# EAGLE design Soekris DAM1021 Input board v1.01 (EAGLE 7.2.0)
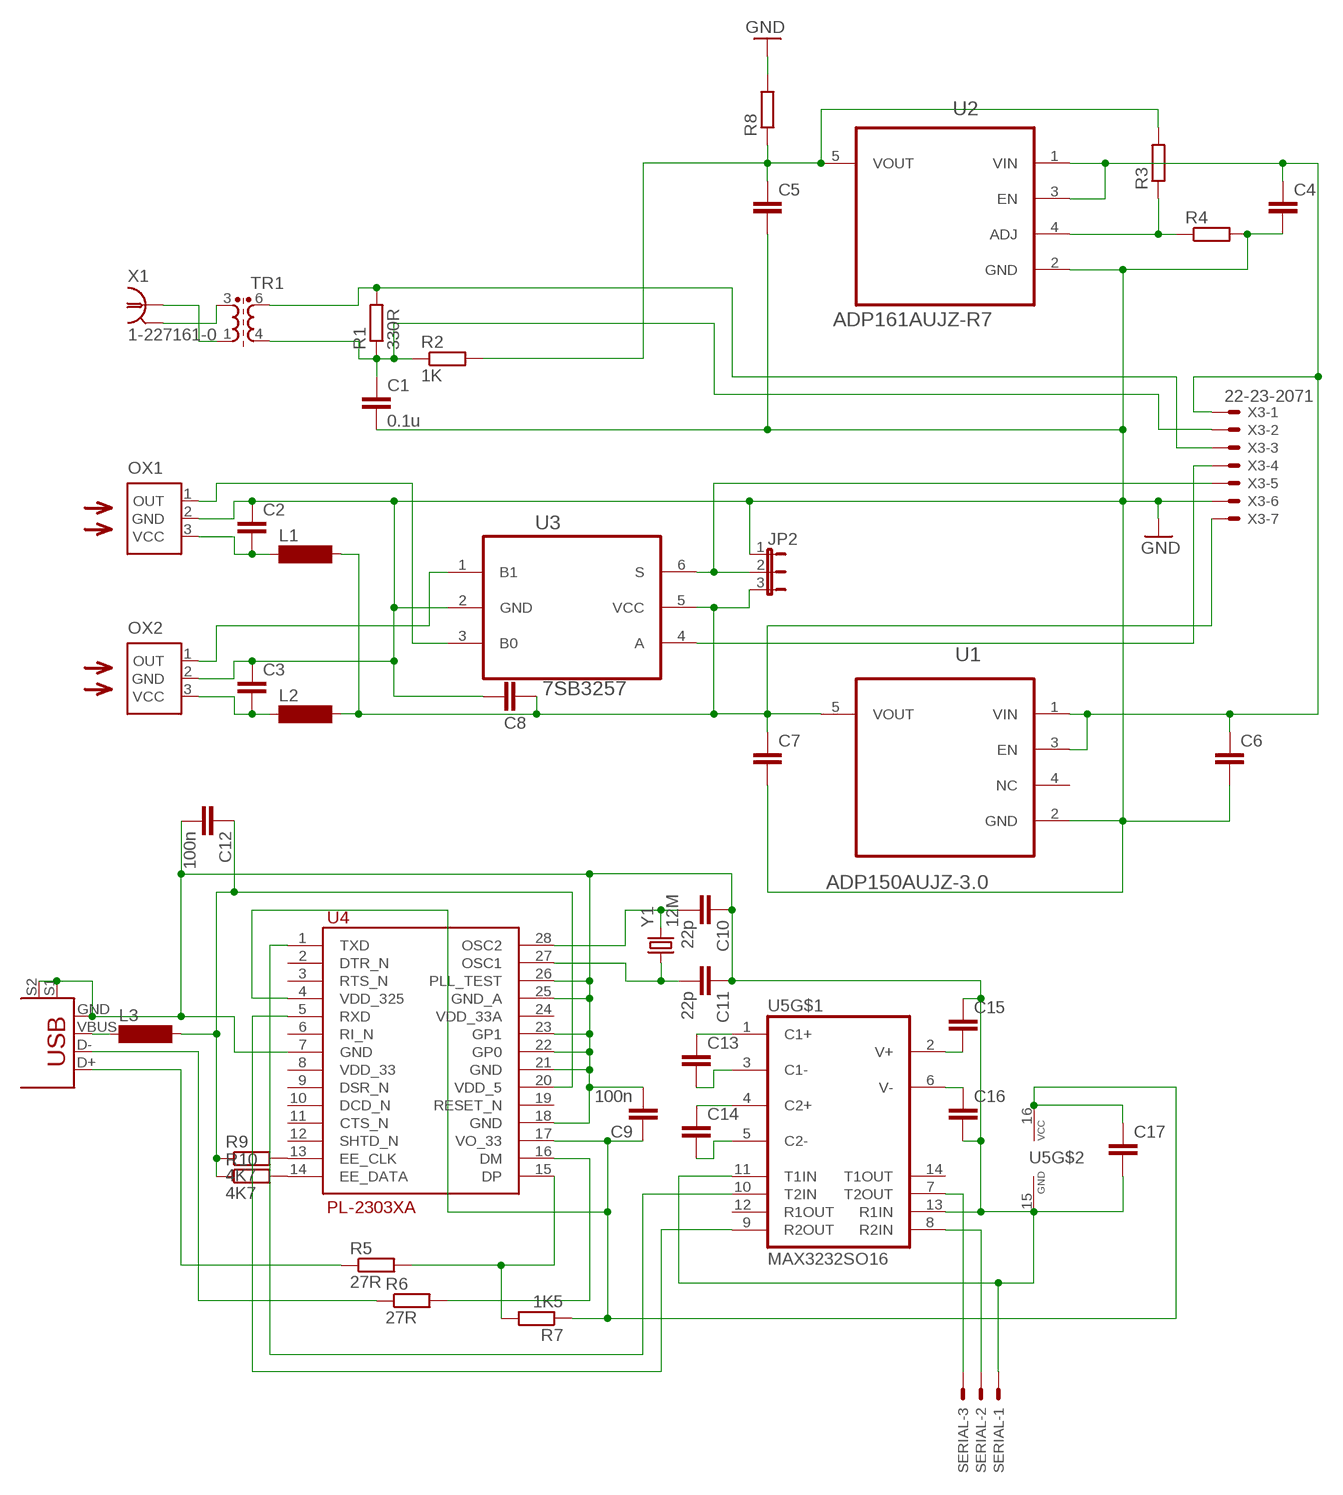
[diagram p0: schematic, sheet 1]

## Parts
C1  0.1u  C-EUC0805  [C0805]
C2  C-EUC0805  [C0805]
C3  C-EUC0805  [C0805]
C4  C-EUC1206  [C1206]
C5  C-EUC1206  [C1206]
C6  C-EUC1206  [C1206]
C7  C-EUC1206  [C1206]
C8  C-EUC1206  [C1206]
C9  100n  C-EUC1206  [C1206]
C10  22p  C-EUC1206  [C1206]
C11  22p  C-EUC1206  [C1206]
C12  100n  C-EUC1206  [C1206]
C13  C-EUC1206  [C1206]
C14  C-EUC1206  [C1206]
C15  C-EUC1206  [C1206]
C16  C-EUC1206  [C1206]
C17  C-EUC1206  [C1206]
JP2  JP2E  [JP2]
L1  SM-1206  [SM-1206]
L2  SM-1206  [SM-1206]
L3  SM-1206  [SM-1206]
OX1  TORX177(F,T)  [TORX]
OX2  TORX177(F,T)  [TORX]
R1  330R  R-EU_R0805  [R0805]
R2  1K  R-EU_R1206  [R1206]
R3  R-EU_R1206  [R1206]
R4  R-EU_R1206  [R1206]
R5  27R  R-EU_M1206  [M1206]
R6  27R  R-EU_M1206  [M1206]
R7  1K5  R-EU_M0805  [M0805]
R8  R-EU_R0805  [R0805]
R9  4K7  R-EU_M0805  [M0805]
R10  4K7  R-EU_M0805  [M0805]
SERIAL  22-23-2031  [22-23-2031]
TR1  DA101C  [DA101C]
U1  ADP150AUJZ-3.0  [SOT95P280X100-5N]
U2  ADP161AUJZ-R7  [SOT95P280X100-5N]
U3  7SB3257  [TSOP-6]
U4  PL-2303XA  [SSOP28]
U5  MAX3232SO16  [SO16]
USB  USB+SHIELD  [USB-B-PTH]
X1  1-227161-0  [AMP_227161]
X3  22-23-2071  [22-23-2071]
Y1  12M  CRYSTALHC49US  [HC49US]

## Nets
GND: C1.2 C2.1 C3.1 C4.2 C5.2 C6.2 C7.2 C8.1 JP2.1 OX1.2(GND) OX2.2(GND) R4.2 R8.2 U1.2(GND) U2.2(GND) U3.2(GND) X3.6
N$1: C4.1 C6.1 U1.1(VIN) U1.3(EN) U2.1(VIN) U2.3(EN) X3.1
N$2: C2.2 L1.1 OX1.3(VCC)
N$3: R3.1 R4.1 U2.4(ADJ)
N$4: C3.2 L2.1 OX2.3(VCC)
N$5: TR1.1 X1.1
N$6: TR1.3 X1.2
N$7: R1.2 TR1.6 X3.3
N$8: C1.1 R1.1 R2.1 TR1.4 X3.2
N$9: C9.1 C17.1 R7.1 U4.4(VDD_325) U4.17(VO_33) U5.16(VCC)
N$10: OX2.1(OUT) U3.1(B1)
N$11: OX1.1(OUT) U3.3(B0)
N$12: C7.1 C8.2 JP2.3 L1.2 L2.2 U1.5(VOUT) U3.5(VCC) X3.7
N$13: JP2.2 U3.6(S) X3.5
N$14: C5.1 R2.2 R3.2 R8.1 U2.5(VOUT)
N$15: R9.2 U4.13(EE_CLK)
N$16: L3.1 USB.VBUS
N$17: U3.4(A) X3.4
N$18: R5.2 R7.2 U4.15(DP)
N$19: R6.2 U4.16(DM)
N$20: R6.1 USB.D-
N$21: R5.1 USB.D+
N$22: C10.2 U4.28(OSC2) Y1.2
N$23: C11.2 U4.27(OSC1) Y1.1
N$24: R10.2 U4.14(EE_DATA)
N$25: C12.1 L3.2 R9.1 R10.1 U4.20(VDD_5)
N$27: SERIAL.2 U5.8(R2IN)
N$28: C13.1 U5.1(C1+)
N$29: C13.2 U5.3(C1-)
N$30: C14.1 U5.4(C2+)
N$31: C14.2 U5.5(C2-)
N$32: C15.2 U5.2(V+)
N$33: C16.1 U5.6(V-)
N$34: C9.2 C10.1 C11.1 C12.2 C15.1 C16.2 C17.2 SERIAL.1 U4.7(GND) U4.18(GND) U4.21(GND) U4.22(GP0) U4.23(GP1) U4.25(GND_A) U4.26(PLL_TEST) U5.11(T1IN) U5.13(R1IN) U5.15(GND2) USB.GND USB.S1 USB.S2
N$37: U4.1(TXD) U5.10(T2IN)
N$38: SERIAL.3 U5.7(T2OUT)
N$40: U4.5(RXD) U5.9(R2OUT)
Unconnected: U1.4(NC) U4.2(DTR_N) U4.3(RTS_N) U4.6(RI_N) U4.8(VDD_33) U4.9(DSR_N) U4.10(DCD_N) U4.11(CTS_N) U4.12(SHTD_N) U4.19(RESET_N) U4.24(VDD_33A) U5.12(R1OUT) U5.14(T1OUT)

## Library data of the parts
C1-C17 = rcl:C-EU: CAPACITOR, European symbol
JP2 = jumper:JP2E: JUMPER
L1-L3 = inductor-neosid:SM-1206: INDUCTOR; OC_FARNELL: unknown; OC_NEWARK: unknown
OX1 OX2 = dir9001_spdif12:TORX177(F,T): FIBER OPTIC RECEIVING MODULE
R1-R10 = rcl:R-EU_: RESISTOR, European symbol
SERIAL = con-molex:22-23-2031: .100" (2.54mm) Center Header - 3 Pin; MF: MOLEX; MPN: 22-23-2031; OC_FARNELL: 1462950; OC_NEWARK: 30C0862
TR1 = Dimdim:DA101C
U1 = Dimdim:ADP150AUJZ-3.0: IC Ultralow Noise,150 mA CMOS Linear Regulator, TSOT-5; MPN: ADP150AUJZ-3.0; OC_FARNELL: 2067776; OC_NEWARK: 73T8165; PACKAGE: TSOT-5; SUPPLIER: Analog Devices
U2 = Dimdim:ADP161AUJZ-R7: 150 mA, CMOS Linear Regulators; MPN: ADP161AUJZ-R7; OC_FARNELL: 2312881; OC_NEWARK: 67W2694; PACKAGE: TSOT-5; SUPPLIER: Analog Devices
U3 = Dimdim:7SB3257
U4 = prolific:PL-2303XA: PL-2303X Edition (Chip Rev A) USB to Serial Bridge Controller (OLD VERSION YEAR 2006) http://www.prolificusa.com/pdf/PL-2303XA.pdf PL-2303X provides a convenient solution for connecting an RS232-like full-duplex asynchronous serial device to any Universal Serial Bus (USB) capable host. PL-2303X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
U5 = maxim-7a:MAX3232SO16
USB = SparkFun-Connectors:USB+SHIELD: USB+Shield USB connector with shield pins connectable
X1 = con-coax-dim:?227161*: JACK, RIGHT ANGLE, 50 OHM, PCB, BNC; MF: TYCO ELECTRONICS; MPN: 1-227161; OC_FARNELL: unknown; OC_NEWARK: 33B3200
X3 = con-molex:22-23-2071: .100" (2.54mm) Center Header - 7 Pin; MF: MOLEX; MPN: 22-23-2071; OC_FARNELL: 1654534; OC_NEWARK: 56H0445
Y1 = SparkFun-FreqCtrl:CRYSTAL: Various standard crystals. Proven footprints.

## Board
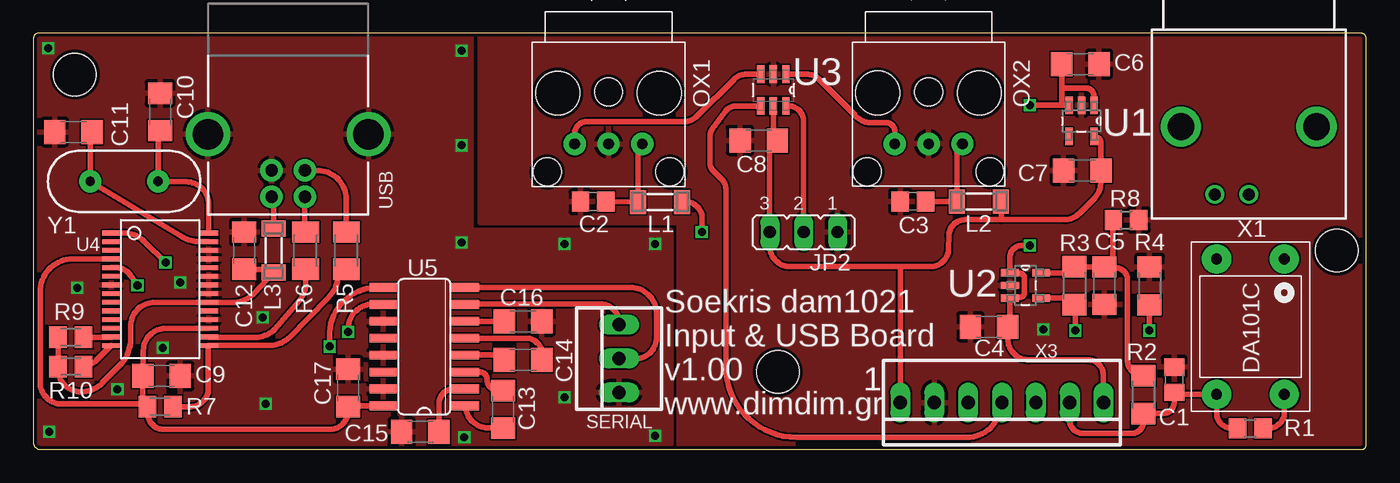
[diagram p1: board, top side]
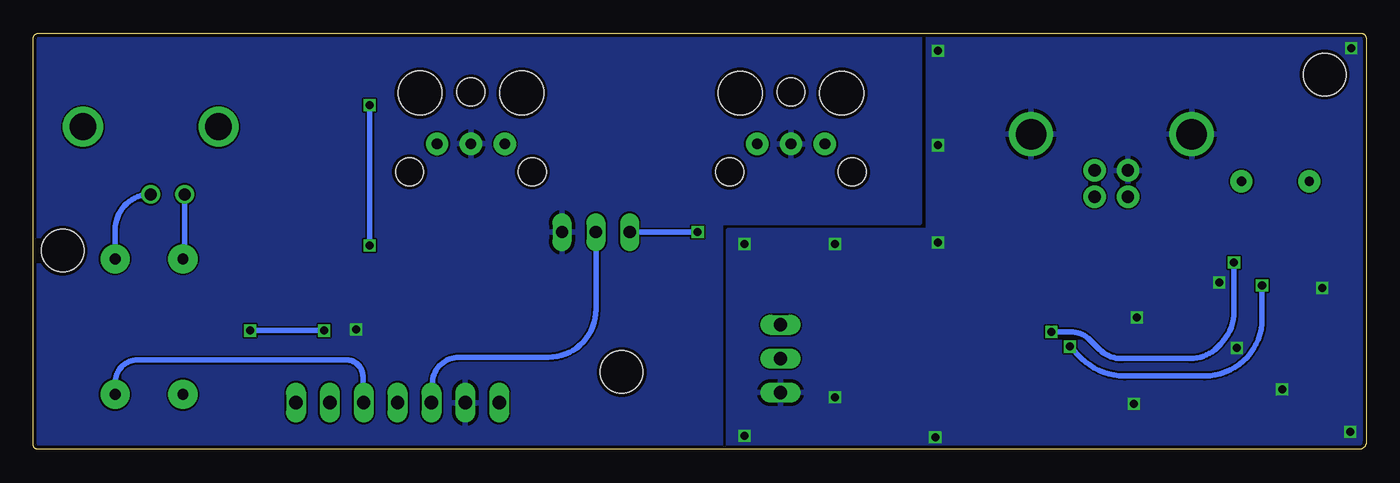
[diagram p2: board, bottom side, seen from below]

Size 99.9 x 31.2 mm. Coordinates in mm from the lower left corner, seen from the top.
Outline: 0,30.78 0,0.56 arc90 0.46,0 99.59,0 arc90 99.9,0.32 99.9,30.84 arc90 99.54,31.2 0.33,31.2 arc90 0,30.78
Copper layers (1*16): Top 0.035mm / dielectric 1.5mm / Bottom 0.035mm
Design rules "dirt_cheap_dirty_boards.v1": minimum track width 5mil, minimum drill 12mil, track to track 5mil, track to pad 5mil, pad to pad 5mil, via to via 5mil, smd to smd 0mil, copper to edge 10mil, drill to drill 10mil, minimum pad ring 10mil, minimum via ring 6mil, stop-mask expansion 2mil, vias tented up to drill 25mil, thermal gap 10mil
Holes 3.2 mm at 3.1,28.1 55.8,5.8 97.7,14.9

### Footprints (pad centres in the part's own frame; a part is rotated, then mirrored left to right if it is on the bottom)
C0805 = smd 1.3 x 1.5: 1 -0.95,0; 2 0.95,0
C1206 = smd 1.6 x 1.8: 1 -1.4,0; 2 1.4,0
JP2 = drill 0.914 long: 1 -2.54,0; 2 0,0; 3 2.54,0
SM-1206 = smd 1.2 x 1.8: 1 -1.65,0; 2 1.65,0
TORX = drill 0.8 pad 1.676: 1 3.81,-2.54; 2 3.81,0; 3 3.81,2.54 | hole 3.3: 0,3.81; 0,-3.81 | hole 2.1: -0.09,0; 5.91,4.6; 5.91,-4.6
R0805 = smd 1.3 x 1.5: 1 -0.95,0; 2 0.95,0
R1206 = smd 1.6 x 1.803: 1 -1.422,0; 2 1.422,0
M1206 = smd 1.6 x 2: 1 -1.4,0; 2 1.4,0
M0805 = smd 1.3 x 1.6: 1 -0.95,0; 2 0.95,0
22-23-2031 = drill 1 long: 1 -2.54,0; 2 0,0; 3 2.54,0
DA101C = drill 0.8 pad 2.184: 1 2.54,5.08; 3 -2.54,5.08; 4 -2.54,-5.08; 6 2.54,-5.08
SOT95P280X100-5N = smd 1.321 x 0.559: 1 -1.168,0.94; 2 -1.168,0; 3 -1.168,-0.94; 4 1.168,-0.94; 5 1.168,0.94
TSOP-6 = smd 1.321 x 0.559: 1 -1.194,2.21; 2 -1.194,1.27; 3 -1.194,0.33; 4 1.194,0.33; 5 1.194,1.27; 6 1.194,2.21
SSOP28 = smd 0.348 x 1.397: 1 -4.225,-3.656; 2 -3.575,-3.656; 3 -2.925,-3.656; 4 -2.275,-3.656; 5 -1.625,-3.656; 6 -0.975,-3.656; 7 -0.325,-3.656; 8 0.325,-3.656; 9 0.975,-3.656; 10 1.625,-3.656; 11 2.275,-3.656; 12 2.925,-3.656; 13 3.575,-3.656; 14 4.225,-3.656; 15 4.225,3.656; 16 3.575,3.656; 17 2.925,3.656; 18 2.275,3.656; 19 1.625,3.656; 20 0.975,3.656; 21 0.325,3.656; 22 -0.325,3.656; 23 -0.975,3.656; 24 -1.625,3.656; 25 -2.275,3.656; 26 -2.925,3.656; 27 -3.575,3.656; 28 -4.225,3.656
SO16 = smd 0.66 x 2.032: 1 -4.445,-3.073; 2 -3.175,-3.073; 3 -1.905,-3.073; 4 -0.635,-3.073; 5 0.635,-3.073; 6 1.905,-3.073; 7 3.175,-3.073; 8 4.445,-3.073; 9 4.445,3.073; 10 3.175,3.073; 11 1.905,3.073; 12 0.635,3.073; 13 -0.635,3.073; 14 -1.905,3.073; 15 -3.175,3.073; 16 -4.445,3.073
USB-B-PTH = drill 0.914 pad 1.676: D+ 0,1.25; D- 1.981,1.25; GND 0,-1.25; VBUS 1.981,-1.25 | drill 2.286: S1 -2.718,-6.02; S2 -2.718,6.02
AMP_227161 = drill 0.9 pad 1.27: 1 0,-5.08; 2 -2.54,-5.08 | drill 2.007: P$1 -5.08,0; P$2 5.08,0
22-23-2071 = drill 1 long: 1 -7.62,0; 2 -5.08,0; 3 -2.54,0; 4 0,0; 5 2.54,0; 6 5.08,0; 7 7.62,0
HC49US = drill 0.7 pad 1.651: 1 -2.54,0; 2 2.54,0

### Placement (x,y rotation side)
C1  85.51,5.22 90 top
C2  41.96,18.58 0 top
C3  65.93,18.59 0 top
C4  71.64,9.19 180 top
C5  80.27,12.27 270 top
C6  78.48,28.89 0 top
C7  78.62,20.92 180 top
C8  54.37,23.17 0 top
C9  9.6,5.5 0 top
C10  9.5,25.3 270 top
C11  3,23.8 0 top
C12  15.8,14.9 90 top
C13  35.2,3 90 top
C14  36.7,6.7 0 top
C15  29,1.3 0 top
C16  36.7,9.6 0 top
C17  23.6,4.6 90 top
JP2  57.74,16.29 180 top
L1  46.96,18.56 0 top
L2  70.88,18.59 0 top
L3  18,14.9 270 top
OX1  43.11,26.71 270 top
OX2  67.1,26.72 270 top
R1  91.21,1.59 0 top
R2  83.2,4.11 90 top
R3  78.03,12.27 90 top
R4  83.66,12.25 90 top
R5  23.46,14.9 270 top
R6  20.4,14.9 270 top
R7  9.5,3.2 0 top
R8  81.9,17.2 0 top
R9  2.8,8.4 0 top
R10  2.8,6.2 0 top
SERIAL  43.9,6.8 90 top
TR1  91.23,9.2 0 top
U1  78.56,24.63 270 top
U2  74.36,12.29 0 top
U3  54.2,26.94 270 top
U4  9.5,12 270 top
U5  29.3,7.7 90 top
USB  19.1,20.92 270 top
X1  91.1,24.2 0 top
X3  72.6,3.5 180 top
Y1  6.8,20.1 0 top

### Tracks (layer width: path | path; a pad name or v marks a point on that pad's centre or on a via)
GND  (via drill 0.6)
  other vias: 75.7,9
  pour Bottom: 33.5,31.2 33.5,17 48.4,17 48.4,0 99.5,-0.1 99.5,31.2
  pour Top: 33.5,31.2 33.5,17 48.4,17 48.4,0 99.5,0 99.5,31.2
N$1  (via drill 0.6)
  Top 0.406: U1.3 77.08,25.8 | 77.08,25.8 77.08,27.1 | 77.08,27.1 C6.1 | U1.1 | U1.1 79.5,26.46 arc90 78.86,27.1 77.08,27.1 | 77.08,25.8 v74.7,25.8 | v74.7,15.3 74.12,15.3 arc90 73.2,14.37 U2.1 73.89,13.21 arc-88 74.3,12.79 74.3,11.81 arc-87 73.9,11.38 U2.3 73.2,9.19 C4.1 73.04,8.28 arc90 74.62,6.7 79.07,6.7 arc-90 80.2,5.57 80.2,3.3 X3.1
  Bottom 0.406: v74.7,25.8 v74.7,15.3
N$2
  Top 0.406: OX1.3 arc37 45.31,22.04 L1.1 C2.2
N$3  (via drill 0.6)
  Top 0.406: U2.4 78.03,11.35 R3.1 78.1,10.85 v78.1,8.9 | R4.1 v83.66,8.9
  Bottom 0.406: v83.66,8.9 v78.1,8.9
N$4
  Top 0.406: OX2.3 69.59,22.88 arc19 69.23,22.18 L2.1 69.09,18.6 C3.2
N$5
  Bottom 0.406: TR1.1 93.77,16.45 arc90 X1.1
N$6
  Bottom 0.406: TR1.3 88.56,14.28 X1.2
N$7
  Top 0.406: TR1.6 93.77,2.53 arc-90 R1.2
  Bottom 0.406: TR1.6 93.77,5.02 arc90 92.09,6.7 76.42,6.7 arc90 75.2,5.48 75.2,3.3 X3.3
N$8
  Top 0.406: 85.5,4.11 C1.1 | C1.1 85.51,4.12 TR1.4 88.69,2.49 arc90 R1.1 | C1.1 85.51,3.51 arc-90 84.69,2.69 R2.1 83.2,2.05 arc-90 82.35,1.2 78.69,1.2 arc-90 77.67,2.21 77.67,3.3 X3.2
N$9
  Top 0.406: U4.17 9.94,9.08 arc89 8.24,7.41 C9.1 8.2,3.55 | 8.2,3.55 R7.1 8.6,3.2 8.6,2.62 arc90 9.72,1.5 22.4,1.5 arc90 C17.1 23.7,3.26 U5.16 | U4.4 2.96,14.28 arc90 0.5,11.82 0.5,5.02 arc90 2.12,3.4 8.2,3.4 8.2,3.55
N$10
  Top 0.406: OX2.1 64.56,23.96 arc90 63.81,24.5 62.59,24.5 arc-45 61.59,25.07 58.94,27.73 arc45 57.95,28.13 U3.1
N$11
  Top 0.406: OX1.1 40.57,23.84 arc-90 41.7,24.56 48.68,24.56 arc45 49.78,25.02 52.5,27.74 arc-45 53.45,28.13 U3.3
N$12  (via drill 0.6)
  Top 0.406: 64.98,13.7 67.24,13.7 arc90 68.6,15.06 68.62,15.97 arc-90 69.83,17.22 72.55,17.23 72.55,17.22 | 64.98,13.7 56.64,13.7 arc-90 55.2,15.34 JP2.3 55.18,16.31 55.18,23.17 C8.2 55.47,23.37 U3.5 | U1.5 arc-90 80.02,22.94 C7.1 80,20.32 80,19.92 arc-45 79.56,18.86 78.39,17.69 arc-45 77.27,17.22 72.55,17.22 | L2.2 72.55,17.22 | L1.2 arc-90 50.1,17.56 v50.1,16.3 | X3.7 64.98,13.7
  Bottom 0.406: JP2.3 v50.1,16.3
N$13
  Top 0.406: U3.6 arc-90 57.74,24.72 JP2.2
  Bottom 0.406: JP2.2 57.74,10.48 arc90 61.32,6.9 67.98,6.9 arc-90 70,4.88 70,3.3 X3.5
N$14
  Top 0.406: U2.5 78.03,13.23 R3.2 80.27,13.69 C5.1 80.27,13.6 80.9,13.6 | R2.2 arc-90 82,6.73 82,12.75 arc90 81.15,13.6 80.9,13.6 | R8.1 80.9,17.1 80.9,13.6
N$15
  Top 0.406: R9.2 5.82,8.4 U4.13
N$16
  Top 0.406: USB.VBUS 18,18.92 L3.1
N$17
  Top 0.406: U3.4 52.66,25.75 arc54 51.87,25.35 50.91,24.04 arc36 50.72,23.47 50.72,21.47 arc45 50.96,20.89 51.65,20.2 arc-45 51.9,19.59 51.9,6.22 arc90 57.22,0.9 70,0.9 arc90 72.5,3.41 | 72.5,3.41 | X3.4 72.6,3.41 72.5,3.41
N$18
  Top 0.406: R5.2 22.9,13.38 arc-44 22.08,11.36 19.2,8.41 arc-46 17.75,7.8 13.18,7.8 U4.15 13.1,7.72 13.1,4.46 arc-45 12.78,3.67 12.64,3.53 arc-45 11.83,3.2 R7.2
N$19
  Top 0.406: R6.2 20.4,12.78 arc-45 19.94,11.14 18.1,9 arc-45 16.65,8.4 13.23,8.4 U4.16
N$20
  Top 0.406: USB.D- 20.35,16.35 R6.1
N$21
  Top 0.406: USB.D+ 21.06,20.9 arc-90 23.44,18.98 R5.1
N$22
  Top 0.406: C10.2 9.34,23.9 Y1.2 11.47,20.07 arc-89 13.15,18.37 U4.28
N$23
  Top 0.406: C11.2 4.26,23.8 Y1.1 11.13,15.95 arc30 12.37,15.59 U4.27
N$24
  Top 0.406: R10.2 3.57,6.2 arc45 4.77,6.69 U4.14
N$25
  Top 0.406: R10.1 R9.1 | C12.1 18.05,13.5 L3.2 16.52,11.66 arc-45 14.97,11.03 U4.20 9.1,11.03 arc90 7.3,9.23 7.3,8.32 arc-45 6.44,6.24 5.18,4.98 arc-45 3.55,4.3 arc-90 1.85,5.99 R10.1 | 1.5,6.2 R10.1
N$27
  Top 0.406: U5.8 44.91,12.14 arc-90 46.7,9.95 46.7,8.36 arc-90 45.14,6.8 SERIAL.2
N$28
  Top 0.406: U5.1 arc90 34.23,1.6 C13.1
N$29
  Top 0.406: U5.3 33.47,5.8 arc-90 34,5.26 arc90 34.86,4.4 C13.2
N$30
  Top 0.406: C14.1 35.34,7.06 U5.4
N$31
  Top 0.406: C14.2 38.2,6.7 arc90 37.07,8.34 U5.5
N$32
  Top 0.406: U5.2 31.51,4.53 arc90 30.4,3.42 C15.2
N$33
  Top 0.406: U5.6 C16.1
N$34  (via drill 0.6)
  other vias: 39.8,3.9 46.6,15.4 32.1,15.5 32.1,29.9 32.1,22.8 39.8,15.4 46.6,1 3.3,12.1 17.2,9.9 9.7,7.6 1.2,1.3 11,12.5 6.3,4.5 32.3,0.9 17.4,3.4 1.1,30.1
  pour Top: -0.1,31.1 32.8,31.1 32.8,16.4 47.8,16.4 47.8,0.4 -0.1,0.2
  pour Bottom: -0.1,31.1 32.8,31.1 32.8,16.4 47.8,16.4 47.8,0.3 -0.1,0.2
N$37  (via drill 0.6)
  Top 0.406: U4.1 6.8,16.23 arc-45 8.3,15.6 v9.9,14 | v23.6,8.8 23.6,8.83 arc-90 25.25,10.88 U5.10
  Bottom 0.406: v9.9,14 9.9,10.36 arc45 10.93,7.87 11.16,7.64 arc45 13.19,6.8 18.3,6.8 arc45 20.01,7.51 20.7,8.2 arc-45 22.15,8.8 v23.6,8.8
N$38
  Top 0.406: U5.7 arc-90 32.7,10.9 42.64,10.9 arc-90 SERIAL.3
N$40  (via drill 0.6)
  Top 0.406: U4.5 6.2,13.62 arc-55 7.27,13.07 v7.8,12.3 | v22.2,7.7 22.2,8.42 arc-90 25.63,12.14 U5.9
  Bottom 0.406: v7.8,12.3 7.8,9.79 arc90 12.1,5.5 18.12,5.5 arc45 21.34,6.83 v22.2,7.7

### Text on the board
tNames: 1 | Soekris dam1021 / Input & USB Board / v1.00 / www.dimdim.gr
